| IBIS file was generated by Viper version: 2022.12.28
[IBIS Ver]   5.0
[Comment Char]   |_char
[File Name]   imxrt700_fowlp324_v1_2.ibs
[File Rev]   1.2
[Date]   Sat Oct 12 16:55:00 2024
[Source]   NXP Viper 2022.12.28
[Notes]
[Disclaimer] IMPORTANT NOTICE
  This information is provided on an AS IS basis and without warranty.
  IN NO EVENT SHALL NXP BE LIABLE FOR INCIDENTAL OR CONSEQUENTIAL
  DAMAGES ARISING FROM USE OF THIS INFORMATION. THIS DISCLAIMER OF
  WARRANTY EXTENDS TO THE USER OF THE INFORMATION, AND TO THEIR CUSTOMERS
  OR USERS OF PRODUCTS  AND IS IN LIEU OF ALL WARRANTIES WHETHER EXPRESS,
  IMPLIED, OR STATUTORY, INCLUDING IMPLIED WARRANTIES OF MERCHANTABILITY
  OR FITNESS FOR PARTICULAR PURPOSE.
  NXP does not represent or warrant that the information furnished
  hereunder is free of infringement of any third party patents,
  copyrights, trade secrets, or other intellectual property rights.
  NXP does not represent or warrant that the information is free of
  defect, or that it meets any particular standard, requirements or need
  of the user of the infomation or their customers.
  NXP reserves the right to change the information in this file
  without notice.
   http://www.nxp.com
[Copyright]   (C) Copyright NXP 2004 - 2024, All Rights Reserved.
|   RT700_324FOWLP_7p3x7p3
[Component]   RT700_324FOWLP_7p3x7p3
[Manufacturer]   NXP
[Package]
| variable   typ   min   max
R_pkg   0.26268   0.033092   0.85076
L_pkg   6.116e-10   1.144e-10   1.896e-09
C_pkg   3.384e-13   6.932e-14   8.387e-13
[Pin] signal_name   model_name   R_pin   L_pin   C_pin
A1   VSS   GND   NA   NA   NA
A2   MIPI_DSI_D1P   mipi   0.25124   1.051e-09 2.160e-13
A3   VSS   GND   NA   NA   NA
A4   MIPI_DSI_D0P   mipi   0.1054   3.119e-10 5.033e-13
A5   VSS   GND   NA   NA   NA
A6   PIO7_9   sd_mmc   0.12364   5.229e-10 1.490e-13
A7   VDDIO_0_4   POWER   NA   NA   NA
A8   VDD2_4   POWER   NA   NA   NA
A9   VDDIO_4   POWER   NA   NA   NA
A10   PIO4_5   sd_mmc   0.21739   8.630e-10 2.078e-13
A11   VSS   GND   NA   NA   NA
A12   VDDIO_4   POWER   NA   NA   NA
A13   VDD1V8   POWER   NA   NA   NA
A14   XTALINSYS   POWER   0.088384  3.992e-10 1.483e-13
A15   VCC18A   POWER   NA   NA   NA
A16   EUSB_DP   NC   0.28532   1.133e-09 1.995e-13
A17   EUSB_DM   NC   0.31827   1.299e-09 2.597e-13
A18   VSS   GND   NA   NA   NA
B1   MIPI_DSI_D1N   mipi   0.24947   1.078e-09 1.747e-13
B2   MIPI_DSI_CLKP   mipi   0.25909   9.091e-10 4.576e-13
B3   MIPI_DSI_CLKN   mipi   0.19446   7.269e-10 4.146e-13
B4   MIPI_DSI_D0N   mipi   0.068162  2.568e-10 2.976e-13
B5   VSS   GND   NA   NA   NA
B6   PIO7_0   sd_mmc   0.048221  3.150e-10 3.099e-13
B7   PIO7_6   sd_mmc   0.066435  1.963e-10 6.932e-14
B8   PIO7_7   sd_mmc   0.062862  3.240e-10 3.793e-13
B9   VDDIO_4   POWER   NA   NA   NA
B10   PIO4_10   sd_mmc   0.071774  2.949e-10 1.133e-13
B11   PIO4_11   sd_mmc   0.068127  3.496e-10 9.386e-14
B12   PIO4_8   sd_mmc   0.05942   3.399e-10 3.223e-13
B13   VDD1V8   POWER   NA   NA   NA
B14   XTALOUTSYS   POWER   0.040514  2.664e-10 2.477e-13
B15   VSS_EUSB   GND   NA   NA   NA
B16   VDD1V2_EUSB   POWER   NA   NA   NA
B17   VSS   GND   NA   NA   NA
B18   USB0_DP   NC   0.18414   6.632e-10 5.281e-13
C1   VDD2_3   POWER   NA   NA   NA
C2   VDD1V8_MIPI   POWER   NA   NA   NA
C3   PIO3_3   sd_mmc   0.20286   5.276e-10 2.379e-13
C4   VDD1V1_MIPI_CAP   POWER   NA   NA   NA
C5   PIO7_11   sd_mmc   0.063089  1.621e-10 3.202e-13
C6   PIO7_8   sd_mmc   0.13739   5.973e-10 3.845e-13
C7   PIO7_1   sd_mmc   0.11529   2.509e-10 1.486e-13
C8   PIO4_6   sd_mmc   0.30677   8.240e-10 4.205e-13
C9   PIO4_4   sd_mmc   0.27533   1.197e-09 5.637e-13
C10   PIO4_3   sd_mmc   0.19226   5.849e-10 3.079e-13
C11   PIO4_2   sd_mmc   0.14036   4.449e-10 2.674e-13
C12   PIO4_9   sd_mmc   0.070802  1.966e-10 1.609e-13
C13   PIO4_7   sd_mmc   0.20436   4.723e-10 3.672e-13
C14   VSSA_1   GND   NA   NA   NA
C15   PIO6_5   sd_mmc   0.11029   2.617e-10 1.678e-13
C16   USB0_VBUS_DETECT   POWER   0.043588  1.679e-10 1.579e-13
C17   VDDN_1   POWER   NA   NA   NA
C18   USB0_DM   NC   0.17462   7.141e-10 4.933e-13
D1   VDDIO_0_3   POWER   NA   NA   NA
D2   PIO3_2   sd_mmc   0.070338  2.788e-10 1.288e-13
D3   PIO2_15   gpiohv   0.20123   4.572e-10 2.051e-13
D4   PIO2_14   gpiohv   0.2838   6.011e-10 2.756e-13
D5   VSS   GND   NA   NA   NA
D6   PIO7_5   sd_mmc   0.13193   2.956e-10 1.907e-13
D7   VSS   GND   NA   NA   NA
D8   PIO4_0   sd_mmc   0.27396   9.004e-10 6.439e-13
D9   PIO4_1   sd_mmc   0.41757   9.862e-10 5.986e-13
D10   PIO4_20   sd_mmc   0.12261   3.165e-10 2.431e-13
D11   VSS   GND   NA   NA   NA
D12   PIO4_19   sd_mmc   0.31578   7.894e-10 4.764e-13
D13   VDDN_1   POWER   NA   NA   NA
D14   PIO6_4   sd_mmc   0.26259   5.271e-10 2.441e-13
D15   PIO6_7   sd_mmc   0.16583   3.647e-10 1.852e-13
D16   PIO6_0   sd_mmc   0.087097  2.313e-10 1.616e-13
D17   PIO6_1   sd_mmc   0.050073  3.030e-10 3.056e-13
D18   VDD3V3_USB   POWER   NA   NA   NA
E1   PIO3_0   sd_mmc   0.095738  4.384e-10 4.933e-13
E2   PIO3_1   sd_mmc   0.073279  1.998e-10 1.005e-13
E3   PIO2_12   gpiohv   0.18394   3.615e-10 3.051e-13
E4   PIO2_13   gpiohv   0.20149   3.491e-10 1.983e-13
E5   PIO7_10   sd_mmc   0.24125   5.709e-10 2.958e-13
E6   PIO7_4   sd_mmc   0.23404   4.870e-10 2.526e-13
E7   VSS   GND   NA   NA   NA
E8   PIO4_13   sd_mmc   0.389   9.169e-10 5.968e-13
E9   PIO4_18   sd_mmc   0.22306   4.870e-10 2.558e-13
E10   PIO4_15   sd_mmc   0.25504   5.203e-10 2.480e-13
E11   VSS   GND   NA   NA   NA
E12   PIO4_14   sd_mmc   0.33868   6.675e-10 4.529e-13
E13   PIO6_6   sd_mmc   0.31661   6.490e-10 4.919e-13
E14   PIO6_10   sd_mmc   0.2699   5.498e-10 2.719e-13
E15   VSS   GND   NA   NA   NA
E16   PIO5_6   sd_mmc   0.087982  1.970e-10 1.469e-13
E17   VDDIO_6   POWER   NA   NA   NA
E18   VDDIO_6   POWER   NA   NA   NA
F1   VDDIO_2   POWER   NA   NA   NA
F2   VDDIO_2   POWER   NA   NA   NA
F3   PIO2_11   gpiohv   0.10106   2.203e-10 1.988e-13
F4   VSS   GND   NA   NA   NA
F5   PIO2_10   gpiohv   0.27823   4.591e-10 4.477e-13
F6   PIO7_3   sd_mmc   0.33143   6.230e-10 3.363e-13
F7   PIO7_2   sd_mmc   0.32068   5.492e-10 3.128e-13
F8   PIO7_12   sd_mmc   0.33209   5.719e-10 4.215e-13
F9   PIO3_11   sd_mmc   0.70515   1.273e-09 5.479e-13
F10   PIO4_16   sd_mmc   0.3   6.269e-10 2.664e-13
F11   PIO4_12   sd_mmc   0.39643   7.821e-10 5.231e-13
F12   PIO4_17   sd_mmc   0.60927   1.113e-09 6.686e-13
F13   PIO6_3   sd_mmc   0.40489   8.103e-10 5.400e-13
F14   PIO6_11   sd_mmc   0.33137   7.151e-10 4.077e-13
F15   PIO6_9   sd_mmc   0.27209   6.555e-10 3.937e-13
F16   PIO5_4   sd_mmc   0.12263   2.688e-10 1.769e-13
F17   PIO5_10   sd_mmc   0.05928   3.299e-10 1.327e-13
F18   PIO5_3   sd_mmc   0.081794  4.401e-10 3.141e-13
G1   PIO2_3   gpiohv   0.10446   4.811e-10 1.576e-13
G2   PIO2_1   gpiohv   0.073468  3.339e-10 3.655e-13
G3   PIO2_4   gpiohv   0.041948  1.249e-10 1.778e-13
G4   PIO2_8   gpiohv   0.18251   2.949e-10 3.065e-13
G5   PIO2_9   gpiohv   0.27427   4.632e-10 3.930e-13
G6   PIO2_7   gpiohv   0.30133   5.353e-10 3.504e-13
G7   PIO3_8   sd_mmc   0.47105   9.259e-10 5.946e-13
G8   PIO3_9   sd_mmc   0.68953   1.205e-09 6.385e-13
G9   PIO3_10   sd_mmc   0.73021   1.279e-09 5.982e-13
G10   PIO6_12   sd_mmc   0.65976   1.205e-09 5.367e-13
G11   PIO6_2   sd_mmc   0.53692   1.044e-09 5.441e-13
G12   PIO7_24   sd_mmc   0.83454   1.421e-09 6.509e-13
G13   PIO6_8   sd_mmc   0.50655   1.022e-09 5.701e-13
G14   VSS   GND   NA   NA   NA
G15   VSS   GND   NA   NA   NA
G16   PIO5_5   sd_mmc   0.15144   4.193e-10 1.904e-13
G17   PIO5_11   sd_mmc   0.061307  2.373e-10 1.100e-13
G18   VSS   GND   NA   NA   NA
H1   VSS   GND   NA   NA   NA
H2   PIO2_0   gpiohv   0.078944  2.644e-10 8.475e-14
H3   PIO2_2   gpiohv   0.097119  2.358e-10 1.325e-13
H4   VSS   GND   NA   NA   NA
H5   VSS   GND   NA   NA   NA
H6   PIO2_6   gpiohv   0.33279   5.774e-10 4.006e-13
H7   PIO3_7   sd_mmc   0.62885   1.108e-09 7.148e-13
H8   VSS   GND   NA   NA   NA
H9   VSS   GND   NA   NA   NA
H10   VSS   GND   NA   NA   NA
H11   VSS   GND   NA   NA   NA
H12   PIO7_25   sd_mmc   0.71492   1.257e-09 5.744e-13
H13   PIO5_0   sd_mmc   0.25927   5.518e-10 3.250e-13
H14   PIO5_18   sd_mmc   0.26524   5.279e-10 2.383e-13
H15   PIO5_13   sd_mmc   0.18785   3.864e-10 2.251e-13
H16   PIO5_8   sd_mmc   0.20506   6.027e-10 2.558e-13
H17   PIO5_1   sd_mmc   0.48674   1.878e-09 4.866e-13
H18   PIO5_2   sd_mmc   0.29709   1.079e-09 2.137e-13
J1   PIO0_0   sd_mmc   0.13849   4.013e-10 4.956e-13
J2   PIO0_1   sd_mmc   0.090132  2.895e-10 1.213e-13
J3   PIO0_2   sd_mmc   0.10694   2.177e-10 1.417e-13
J4   PIO0_3   sd_mmc   0.21035   3.934e-10 2.174e-13
J5   PIO0_6   sd_mmc   0.2925   5.111e-10 2.939e-13
J6   PIO2_5   gpiohv   0.40854   6.791e-10 4.359e-13
J7   PIO3_6   sd_mmc   0.6273   1.093e-09 7.327e-13
J8   VSS   GND   NA   NA   NA
J9   VSS   GND   NA   NA   NA
J10   VSS   GND   NA   NA   NA
J11   VSS   GND   NA   NA   NA
J12   PIO8_26   gpio   0.75268   1.293e-09 6.117e-13
J13   PIO8_25   gpio   0.85076   1.583e-09 8.387e-13
J14   PIO5_15   sd_mmc   0.32094   7.312e-10 4.968e-13
J15   PIO5_16   sd_mmc   0.16604   4.852e-10 3.898e-13
J16   PIO5_9   sd_mmc   0.43442   1.046e-09 4.435e-13
J17   VDDIO_5   POWER   NA   NA   NA
J18   VDDIO_5   POWER   NA   NA   NA
K1   VDD2_2   POWER   NA   NA   NA
K2   VDD2_2   POWER   NA   NA   NA
K3   PIO0_5   sd_mmc   0.13395   3.094e-10 1.725e-13
K4   PIO0_4   sd_mmc   0.18653   3.791e-10 2.301e-13
K5   PIO0_7   sd_mmc   0.26742   5.072e-10 2.779e-13
K6   PIO3_4   sd_mmc   0.68031   1.153e-09 7.735e-13
K7   PIO3_5   sd_mmc   0.74255   1.238e-09 8.110e-13
K8   VSS   GND   NA   NA   NA
K9   VSS   GND   NA   NA   NA
K10   VSS   GND   NA   NA   NA
K11   VSS   GND   NA   NA   NA
K12   PIO8_27   gpio   0.65334   1.167e-09 5.593e-13
K13   PIO5_17   sd_mmc   0.3988   8.762e-10 4.868e-13
K14   PIO5_20   sd_mmc   0.35477   7.846e-10 4.492e-13
K15   PIO5_12   sd_mmc   0.23943   7.581e-10 3.363e-13
K16   PIO5_7   sd_mmc   0.35528   1.896e-09 4.801e-13
K17   PIO7_22   sd_mmc   0.059205  3.037e-10 3.223e-13
K18   PIO7_21   sd_mmc   0.088293  4.583e-10 3.666e-13
L1   PIO0_14   sd_mmc   0.11544   4.719e-10 1.283e-13
L2   PIO0_15   sd_mmc   0.066923  2.679e-10 1.285e-13
L3   PIO0_13   sd_mmc   0.094025  2.185e-10 1.477e-13
L4   PIO0_11   sd_mmc   0.16333   3.153e-10 2.063e-13
L5   PIO0_12   sd_mmc   0.26198   4.735e-10 3.649e-13
L6   PIO0_10   sd_mmc   0.34512   6.036e-10 4.896e-13
L7   PIO0_9   sd_mmc   0.41862   7.057e-10 5.931e-13
L8   VSS   GND   NA   NA   NA
L9   VSS   GND   NA   NA   NA
L10   VSS   GND   NA   NA   NA
L11   VSS   GND   NA   NA   NA
L12   PIO8_28   gpio   0.6211   1.126e-09 5.261e-13
L13   PIO5_19   sd_mmc   0.51582   1.825e-09 5.851e-13
L14   VSS   GND   NA   NA   NA
L15   VSS   GND   NA   NA   NA
L16   PIO7_18   sd_mmc   0.12585   2.973e-10 2.004e-13
L17   PIO7_17   sd_mmc   0.090307  5.404e-10 2.800e-13
L18   VDD2_0   POWER   NA   NA   NA
M1   VDDIO_0_2   POWER   NA   NA   NA
M2   PIO0_21   sd_mmc   0.064707  2.950e-10 3.688e-13
M3   PIO0_22   sd_mmc   0.099218  2.143e-10 9.874e-14
M4   VSS   GND   NA   NA   NA
M5   VSS   GND   NA   NA   NA
M6   PIO0_16   sd_mmc   0.34114   5.716e-10 4.635e-13
M7   PIO0_18   sd_mmc   0.51145   8.514e-10 4.167e-13
M8   PIO0_19   sd_mmc   0.53104   8.685e-10 5.914e-13
M9   PIO0_20   sd_mmc   0.65857   1.065e-09 7.339e-13
M10   PIO10_16   gpio   0.74355   1.222e-09 7.746e-13
M11   PIO10_15   gpio   0.70048   1.171e-09 6.645e-13
M12   PIO10_14   gpio   0.55175   1.004e-09 4.267e-13
M13   PIO5_14   sd_mmc   0.79821   1.373e-09 6.326e-13
M14   PIO7_15   sd_mmc   0.36129   7.960e-10 3.382e-13
M15   PIO7_16   sd_mmc   0.32048   8.596e-10 3.203e-13
M16   PIO8_7   gpio   0.11214   2.506e-10 1.514e-13
M17   PIO7_19   sd_mmc   0.12933   8.259e-10 2.940e-13
M18   PIO7_20   sd_mmc   0.14795   6.174e-10 1.476e-13
N1   PIO1_8   sd_mmc   0.19503   4.539e-10 2.024e-13
N2   PIO1_6   sd_mmc   0.16869   3.842e-10 5.100e-13
N3   PIO1_7   sd_mmc   0.223   5.144e-10 2.946e-13
N4   PIO0_31   sd_mmc   0.2088   3.681e-10 3.451e-13
N5   PIO1_0   sd_mmc   0.24232   4.470e-10 3.909e-13
N6   PIO0_17   sd_mmc   0.42268   7.407e-10 5.357e-13
N7   PMIC_MODE0   reset   0.71141   1.146e-09 5.418e-13
N8   PMIC_IRQN   gpio   0.61893   1.045e-09 4.873e-13
N9   PIO8_22   gpio   0.42049   7.439e-10 4.711e-13
N10   PIO10_17   gpio   0.72932   1.225e-09 7.125e-13
N11   PIO8_11   gpio   0.37601   6.916e-10 3.223e-13
N12   PIO8_10   gpio   0.38915   8.111e-10 3.420e-13
N13   PIO8_9   gpio   0.32668   6.628e-10 3.350e-13
N14   PIO7_23   sd_mmc   0.39583   9.471e-10 5.739e-13
N15   VSS   GND   NA   NA   NA
N16   PIO8_23   gpio   0.081719  4.063e-10 3.349e-13
N17   VDDIO_0_0   POWER   NA   NA   NA
N18   VDDIO_0_0   POWER   NA   NA   NA
P1   VSS   GND   NA   NA   NA
P2   VSS   GND   NA   NA   NA
P3   PIO1_14   sd_mmc   0.23155   4.677e-10 2.125e-13
P4   VSS   GND   NA   NA   NA
P5   PIO1_16   sd_mmc   0.22183   4.261e-10 2.054e-13
P6   PIO1_3   sd_mmc   0.28608   5.238e-10 3.286e-13
P7   PIO1_19   sd_mmc   0.41468   7.481e-10 3.525e-13
P8   VSS   GND   NA   NA   NA
P9   PIO8_19   gpio   0.32192   6.199e-10 3.699e-13
P10   PIO8_18   gpio   0.28934   5.565e-10 2.656e-13
P11   PIO8_12   gpio   0.33499   6.014e-10 4.740e-13
P12   VSS   GND   NA   NA   NA
P13   PIO8_30   gpio   0.32292   6.969e-10 3.223e-13
P14   PIO7_14   sd_mmc   0.35818   9.088e-10 3.617e-13
P15   PIO7_13   sd_mmc   0.28238   8.133e-10 3.868e-13
P16   PIO8_24   gpio   0.13641   3.373e-10 2.519e-13
P17   PIO10_3   gpio   0.10987   3.324e-10 3.455e-13
P18   PIO10_2   gpio   0.10227   5.228e-10 3.512e-13
R1   PIO1_12   sd_mmc   0.13573   5.705e-10 1.736e-13
R2   PIO1_11   sd_mmc   0.12126   5.284e-10 1.544e-13
R3   PIO1_13   sd_mmc   0.099978  2.118e-10 1.234e-13
R4   PIO1_17   sd_mmc   0.16732   3.573e-10 1.848e-13
R5   PIO1_18   sd_mmc   0.24552   4.548e-10 2.470e-13
R6   VSS   GND   NA   NA   NA
R7   PMIC_MODE1   reset   0.5507   8.938e-10 4.397e-13
R8   VSS   GND   NA   NA   NA
R9   PIO8_21   gpio   0.26922   5.156e-10 2.796e-13
R10   PIO8_14   gpio   0.26762   5.082e-10 2.516e-13
R11   PIO8_13   gpio   0.25   4.644e-10 2.232e-13
R12   VSS   GND   NA   NA   NA
R13   PIO8_31   gpio   0.33217   7.658e-10 3.659e-13
R14   VSS   GND   NA   NA   NA
R15   PIO10_4   gpio   0.12844   2.670e-10 2.052e-13
R16   PIO10_5   gpio   0.14117   3.322e-10 1.931e-13
R17   PIO10_0   gpio   0.085361  2.202e-10 3.274e-13
R18   VSS   GND   NA   NA   NA
T1   VDDIO_0_2   POWER   NA   NA   NA
T2   PIO1_10   sd_mmc   0.056962  2.821e-10 8.327e-14
T3   PIO1_5   sd_mmc   0.10396   2.135e-10 2.479e-13
T4   PIO1_4   sd_mmc   0.19114   3.228e-10 2.658e-13
T5   PIO1_9   sd_mmc   0.25441   4.057e-10 2.632e-13
T6   PIO1_15   sd_mmc   0.41215   7.309e-10 3.938e-13
T7   PIO1_2   sd_mmc   0.51869   9.147e-10 3.976e-13
T8   PIO8_20   gpio   0.28851   5.926e-10 3.523e-13
T9   PIO8_16   gpio   0.17418   3.140e-10 3.282e-13
T10   PIO8_15   gpio   0.096143  2.258e-10 2.472e-13
T11   PIO8_8   gpio   0.15183   3.244e-10 2.030e-13
T12   PIO8_1   gpio   0.15057   3.139e-10 1.938e-13
T13   PIO8_6   gpio   0.033092  1.144e-10 1.391e-13
T14   PIO10_6   gpio   0.11141   2.330e-10 1.541e-13
T15   PIO10_7   gpio   0.11856   2.511e-10 1.740e-13
T16   VREF_LDO   POWER   NA   NA   NA
T17   PIO10_1   gpio   0.089893  2.334e-10 4.163e-13
T18   PIO10_9   gpio   0.1209   3.477e-10 1.835e-13
U1   VDDIO_AO   POWER   NA   NA   NA
U2   VSS   GND   NA   NA   NA
U3   RESETN   reset   0.11889   2.360e-10 1.685e-13
U4   VDD1V8_AO   POWER   NA   NA   NA
U5   VDDN_0   POWER   NA   NA   NA
U6   VDD2_1   POWER   NA   NA   NA
U7   PMIC_I2C_SDA   gpio   0.1036   6.928e-10 4.221e-13
U8   PMIC_I2C_SCL   gpio   0.16925   9.938e-10 1.593e-13
U9   PIO8_17   gpio   0.22635   8.227e-10 5.004e-13
U10   VDD1   POWER   NA   NA   NA
U11   PIO8_2   gpio   0.10607   5.637e-10 4.373e-13
U12   PIO8_0   gpio   0.067902  2.438e-10 7.663e-14
U13   PIO8_5   gpio   0.067019  2.004e-10 3.449e-13
U14   VDDIO_0_1   POWER   NA   NA   NA
U15   PIO10_12   gpio   0.072742  3.968e-10 1.426e-13
U16   VREFH_ANA18   POWER   NA   NA   NA
U17   VREFL_ANA   POWER   NA   NA   NA
U18   PIO10_8   gpio   0.12168   3.775e-10 1.372e-13
V1   VSS   GND   NA   NA   NA
V2   XTALIN32KHZ   POWER   0.20791   1.009e-09 2.303e-13
V3   XTALOUT32KHZ   POWER   0.20324   6.472e-10 2.165e-13
V4   VDD1V8_AO   POWER   NA   NA   NA
V5   VSS   GND   NA   NA   NA
V6   VDD2_1   POWER   NA   NA   NA
V7   VDD1V8_DCDC   POWER   NA   NA   NA
V8   LX_DCDC   NC   0.034441  3.259e-10 3.584e-13
V9   VSS_DCDC   GND   NA   NA   NA
V10   VDD1   POWER   NA   NA   NA
V11   PIO8_3   gpio   0.11538   5.836e-10 1.100e-13
V12   VSS   GND   NA   NA   NA
V13   PIO8_4   gpio   0.11654   4.759e-10 2.414e-13
V14   VDDIO_0_1   POWER   NA   NA   NA
V15   PIO10_13   gpio   0.10932   5.018e-10 1.214e-13
V16   VDDA_1V8   POWER   NA   NA   NA
V17   VSSA_0   GND   NA   NA   NA
V18   VSSA_0   GND   NA   NA   NA
[Pin Mapping]   pulldown_ref   pullup_ref
A1   VSS   NC
A2   VSS   VDD1V8_MIPI
A3   VSS   NC
A4   VSS   VDD1V8_MIPI
A5   VSS   NC
A6   VSS   NC
A7   NC   VDDIO_0_4
A8   NC   VDD2_4
A9   NC   VDDIO_4
A10   VSS   VDDIO_4
A11   VSS   NC
A12   NC   VDDIO_4
A13   NC   VDD1V8
A14   NC   VDD1V8
A15   NC   VCC18A
A16   NC   NC
A17   NC   NC
A18   VSS   NC
B1   VSS   VDD1V8_MIPI
B2   VSS   VDD1V8_MIPI
B3   VSS   VDD1V8_MIPI
B4   VSS   VDD1V8_MIPI
B5   VSS   NC
B6   VSS   NC
B7   VSS   NC
B8   VSS   NC
B9   NC   VDDIO_4
B10   VSS   VDDIO_4
B11   VSS   VDDIO_4
B12   VSS   VDDIO_4
B13   NC   VDD1V8
B14   NC   VDD1V8
B15   VSS   NC
B16   NC   VDD1V2_EUSB
B17   VSS   NC
B18   NC   NC
C1   NC   VDD2_3
C2   NC   VDD1V8_MIPI
C3   VSS   NC
C4   NC   VDD1V1_MIPI_CAP
C5   VSS   NC
C6   VSS   NC
C7   VSS   NC
C8   VSS   VDDIO_4
C9   VSS   VDDIO_4
C10   VSS   VDDIO_4
C11   VSS   VDDIO_4
C12   VSS   VDDIO_4
C13   VSS   VDDIO_4
C14   VSSA_1   NC
C15   VSS   VDDIO_6
C16   NC   VDD3V3_USB
C17   NC   VDDN_1
C18   NC   NC
D1   NC   VDDIO_0_3
D2   VSS   NC
D3   VSS   VDDIO_2
D4   VSS   VDDIO_2
D5   VSS   NC
D6   VSS   NC
D7   VSS   NC
D8   VSS   VDDIO_4
D9   VSS   VDDIO_4
D10   VSS   VDDIO_4
D11   VSS   NC
D12   VSS   VDDIO_4
D13   NC   VDDN_1
D14   VSS   VDDIO_6
D15   VSS   VDDIO_6
D16   VSS   VDDIO_6
D17   VSS   VDDIO_6
D18   NC   VDD3V3_USB
E1   VSS   NC
E2   VSS   NC
E3   VSS   VDDIO_2
E4   VSS   VDDIO_2
E5   VSS   NC
E6   VSS   NC
E7   VSS   NC
E8   VSS   VDDIO_4
E9   VSS   VDDIO_4
E10   VSS   VDDIO_4
E11   VSS   NC
E12   VSS   VDDIO_4
E13   VSS   VDDIO_6
E14   VSS   VDDIO_6
E15   VSS   NC
E16   VSS   VDDIO_5
E17   NC   VDDIO_6
E18   NC   VDDIO_6
F1   NC   VDDIO_2
F2   NC   VDDIO_2
F3   VSS   VDDIO_2
F4   VSS   NC
F5   VSS   VDDIO_2
F6   VSS   NC
F7   VSS   NC
F8   VSS   NC
F9   VSS   NC
F10   VSS   VDDIO_4
F11   VSS   VDDIO_4
F12   VSS   VDDIO_4
F13   VSS   VDDIO_6
F14   VSS   VDDIO_6
F15   VSS   VDDIO_6
F16   VSS   VDDIO_5
F17   VSS   VDDIO_5
F18   VSS   VDDIO_5
G1   VSS   VDDIO_2
G2   VSS   VDDIO_2
G3   VSS   VDDIO_2
G4   VSS   VDDIO_2
G5   VSS   VDDIO_2
G6   VSS   VDDIO_2
G7   VSS   NC
G8   VSS   NC
G9   VSS   NC
G10   VSS   VDDIO_6
G11   VSS   VDDIO_6
G12   VSS   NC
G13   VSS   VDDIO_6
G14   VSS   NC
G15   VSS   NC
G16   VSS   VDDIO_5
G17   VSS   VDDIO_5
G18   VSS   NC
H1   VSS   NC
H2   VSS   VDDIO_2
H3   VSS   VDDIO_2
H4   VSS   NC
H5   VSS   NC
H6   VSS   VDDIO_2
H7   VSS   NC
H8   VSS   NC
H9   VSS   NC
H10   VSS   NC
H11   VSS   NC
H12   VSS   NC
H13   VSS   VDDIO_5
H14   VSS   VDDIO_5
H15   VSS   VDDIO_5
H16   VSS   VDDIO_5
H17   VSS   VDDIO_5
H18   VSS   VDDIO_5
J1   VSS   NC
J2   VSS   NC
J3   VSS   NC
J4   VSS   NC
J5   VSS   NC
J6   VSS   VDDIO_2
J7   VSS   NC
J8   VSS   NC
J9   VSS   NC
J10   VSS   NC
J11   VSS   NC
J12   VSS   NC
J13   VSS   NC
J14   VSS   VDDIO_5
J15   VSS   VDDIO_5
J16   VSS   VDDIO_5
J17   NC   VDDIO_5
J18   NC   VDDIO_5
K1   NC   VDD2_2
K2   NC   VDD2_2
K3   VSS   NC
K4   VSS   NC
K5   VSS   NC
K6   VSS   NC
K7   VSS   NC
K8   VSS   NC
K9   VSS   NC
K10   VSS   NC
K11   VSS   NC
K12   VSS   NC
K13   VSS   VDDIO_5
K14   VSS   VDDIO_5
K15   VSS   VDDIO_5
K16   VSS   VDDIO_5
K17   VSS   NC
K18   VSS   NC
L1   VSS   NC
L2   VSS   NC
L3   VSS   NC
L4   VSS   NC
L5   VSS   NC
L6   VSS   NC
L7   VSS   NC
L8   VSS   NC
L9   VSS   NC
L10   VSS   NC
L11   VSS   NC
L12   VSS   NC
L13   VSS   VDDIO_5
L14   VSS   NC
L15   VSS   NC
L16   VSS   NC
L17   VSS   NC
L18   NC   VDD2_0
M1   NC   VDDIO_0_2
M2   VSS   NC
M3   VSS   NC
M4   VSS   NC
M5   VSS   NC
M6   VSS   NC
M7   VSS   NC
M8   VSS   NC
M9   VSS   NC
M10   VSS   NC
M11   VSS   NC
M12   VSS   NC
M13   VSS   VDDIO_5
M14   VSS   NC
M15   VSS   NC
M16   VSS   NC
M17   VSS   NC
M18   VSS   NC
N1   VSS   NC
N2   VSS   NC
N3   VSS   NC
N4   VSS   NC
N5   VSS   NC
N6   VSS   NC
N7   VSS   VDDIO_AO
N8   VSS   VDDIO_AO
N9   VSS   NC
N10   VSS   NC
N11   VSS   NC
N12   VSS   NC
N13   VSS   NC
N14   VSS   NC
N15   VSS   NC
N16   VSS   NC
N17   NC   VDDIO_0_0
N18   NC   VDDIO_0_0
P1   VSS   NC
P2   VSS   NC
P3   VSS   NC
P4   VSS   NC
P5   VSS   NC
P6   VSS   NC
P7   VSS   NC
P8   VSS   NC
P9   VSS   NC
P10   VSS   NC
P11   VSS   NC
P12   VSS   NC
P13   VSS   NC
P14   VSS   NC
P15   VSS   NC
P16   VSS   NC
P17   VSS   NC
P18   VSS   NC
R1   VSS   NC
R2   VSS   NC
R3   VSS   NC
R4   VSS   NC
R5   VSS   NC
R6   VSS   NC
R7   VSS   VDDIO_AO
R8   VSS   NC
R9   VSS   NC
R10   VSS   NC
R11   VSS   NC
R12   VSS   NC
R13   VSS   NC
R14   VSS   NC
R15   VSS   NC
R16   VSS   NC
R17   VSS   NC
R18   VSS   NC
T1   NC   VDDIO_0_2
T2   VSS   NC
T3   VSS   NC
T4   VSS   NC
T5   VSS   NC
T6   VSS   NC
T7   VSS   NC
T8   VSS   NC
T9   VSS   NC
T10   VSS   NC
T11   VSS   NC
T12   VSS   NC
T13   VSS   NC
T14   VSS   NC
T15   VSS   NC
T16   NC   VDDA_1V8
T17   VSS   NC
T18   VSS   NC
U1   NC   VDDIO_AO
U2   VSS   NC
U3   VSS   VDDIO_AO
U4   NC   VDD1V8_AO
U5   NC   VDDN_0
U6   NC   VDD2_1
U7   VSS   NC
U8   VSS   NC
U9   VSS   NC
U10   NC   VDD1
U11   VSS   NC
U12   VSS   NC
U13   VSS   NC
U14   NC   VDDIO_0_1
U15   VSS   NC
U16   NC   VDDA_1V8
U17   NC   VDDA_1V8
U18   VSS   NC
V1   VSS   NC
V2   NC   VDDIO_AO
V3   NC   VDDIO_AO
V4   NC   VDD1V8_AO
V5   VSS   NC
V6   NC   VDD2_1
V7   NC   VDD1V8_DCDC
V8   NC   NC
V9   VSS_DCDC   NC
V10   NC   VDD1
V11   VSS   NC
V12   VSS   NC
V13   VSS   NC
V14   NC   VDDIO_0_1
V15   VSS   NC
V16   NC   VDDA_1V8
V17   VSSA_0   NC
V18   VSSA_0   NC
[Diff Pin]  inv_pin  vdiff  tdelay_typ tdelay_min tdelay_max
A2   B1   NA   NA   NA   NA
A4   B4   NA   NA   NA   NA
B2   B3   NA   NA   NA   NA
|*   Model Selector   *
[Model Selector] gpio
io_crdrobe1dse0sre0   Derated range in cont mode, 5mA drive strength, without slew rate
io_crdrobe1dse0sre1   Derated range in cont mode, 5mA drive strength, with slew rate
io_crdrobe1dse1sre0   Derated range in cont mode, 10mA drive strength, without slew rate
io_crdrobe1dse1sre1   Derated range in cont mode, 10mA drive strength, with slew rate
io_crdr2obe1dse0sre0   Derated2 range in cont mode, 5mA drive strength, without slew rate
io_crdr2obe1dse0sre1   Derated2 range in cont mode, 5mA drive strength, with slew rate
io_crdr2obe1dse1sre0   Derated2 range in cont mode, 10mA drive strength, without slew rate
io_crdr2obe1dse1sre1   Derated2 range in cont mode, 10mA drive strength, with slew rate
io_lrobe1dse0sre0   low range mode, 5mA drive strength, without slew rate
io_lrobe1dse0sre1   low range mode, 5mA drive strength, with slew rate
io_lrobe1dse1sre0   low range mode, 10mA drive strength, without slew rate
io_lrobe1dse1sre1   low range mode, 10mA drive strength, with slew rate
[Model Selector] gpiohv
io_crnrobe1dse0sre0   Normal range in cont mode, 5mA drive strength, without slew rate
io_crnrobe1dse0sre1   Normal range in cont mode, 5mA drive strength, with slew rate
io_crnrobe1dse1sre0   Normal range in cont mode, 10mA drive strength, without slew rate
io_crnrobe1dse1sre1   Normal range in cont mode, 10mA drive strength, with slew rate
io_crdrobe1dse0sre0   Derated range in cont mode, 5mA drive strength, without slew rate
io_crdrobe1dse0sre1   Derated range in cont mode, 5mA drive strength, with slew rate
io_crdrobe1dse1sre0   Derated range in cont mode, 10mA drive strength, without slew rate
io_crdrobe1dse1sre1   Derated range in cont mode, 10mA drive strength, with slew rate
io_crdr2obe1dse0sre0   Derated2 range in cont mode, 5mA drive strength, without slew rate
io_crdr2obe1dse0sre1   Derated2 range in cont mode, 5mA drive strength, with slew rate
io_crdr2obe1dse1sre0   Derated2 range in cont mode, 10mA drive strength, without slew rate
io_crdr2obe1dse1sre1   Derated2 range in cont mode, 10mA drive strength, with slew rate
io_hrobe1dse0sre0   high range mode, 5mA drive strength, without slew rate
io_hrobe1dse0sre1   high range mode, 5mA drive strength, with slew rate
io_hrobe1dse1sre0   high range mode, 10mA drive strength, without slew rate
io_hrobe1dse1sre1   high range mode, 10mA drive strength, with slew rate
io_lrobe1dse0sre0   low range mode, 5mA drive strength, without slew rate
io_lrobe1dse0sre1   low range mode, 5mA drive strength, with slew rate
io_lrobe1dse1sre0   low range mode, 10mA drive strength, without slew rate
io_lrobe1dse1sre1   low range mode, 10mA drive strength, with slew rate
io_crnrobe1dse0sre0_5pct   Narrow range in cont mode, 5mA drive strength, without slew rate
io_crnrobe1dse0sre1_5pct   Narrow range in cont mode, 5mA drive strength, with slew rate
io_crnrobe1dse1sre0_5pct   Narrow range in cont mode, 10mA drive strength, without slew rate
io_crnrobe1dse1sre1_5pct   Narrow range in cont mode, 10mA drive strength, with slew rate
io_hrobe1dse0sre0_5pct   Narrow range in high range mode, 5mA drive strength, without slew rate
io_hrobe1dse0sre1_5pct   Narrow range in high range mode, 5mA drive strength, with slew rate
io_hrobe1dse1sre0_5pct   Narrow range in high range mode, 10mA drive strength, without slew rate
io_hrobe1dse1sre1_5pct   Narrow range in high range mode, 10mA drive strength, with slew rate
[Model Selector] mipi
MIPI_HS   MIPI DSI High Speed Mode
MIPI_LP   MIPI DSI Low Power Mode
[Model Selector] reset
io_rst_crdrobe1dse0sre0   Derated voltage range in cont mode, 5mA current drive strength, without slew rate
io_rst_crdrobe1dse0sre1   Derated voltage range in cont mode, 5mA current drive strength, with slew rate
io_rst_crdrobe1dse1sre0   Derated voltage range in cont mode, 10mA current drive strength, without slew rate
io_rst_crdrobe1dse1sre1   Derated voltage range in cont mode, 10mA current drive strength, with slew rate
io_rst_crdr2obe1dse0sre0   Derated2 voltage range in cont mode, 5mA current drive strength, without slew rate
io_rst_crdr2obe1dse0sre1   Derated2 voltage range in cont mode, 5mA current drive strength, with slew rate
io_rst_crdr2obe1dse1sre0   Derated2 voltage range in cont mode, 10mA current drive strength, without slew rate
io_rst_crdr2obe1dse1sre1   Derated2 voltage range in cont mode, 10mA current drive strength, with slew rate
io_rst_lrobe1dse0sre0   low range mode, 5mA current drive strength, without slew rate
io_rst_lrobe1dse0sre1   low range mode, 5mA current drive strength, with slew rate
io_rst_lrobe1dse1sre0   low range mode, 10mA current drive strength, without slew rate
io_rst_lrobe1dse1sre1   low range mode, 10mA current drive strength, with slew rate
[Model Selector] sd_mmc
io_nvldro0drz0   Normal voltage level DRIVE1=0 DRIVE0=0 1.8v voltage domain function mode with 100ohm transmitter drive
io_nvldro0drz1   Normal voltage level DRIVE1=0 DRIVE0=1 1.8v voltage domain function mode with 66ohm transmitter drive
io_nvldro1drz0   Normal voltage level DRIVE1=1 DRIVE0=0 1.8v voltage domain function mode with 50ohm transmitter drive
io_nvldro1drz1   Normal voltage level DRIVE1=1 DRIVE0=1 1.8v voltage domain function mode with 33ohm transmitter drive
io_lvldro0drz0   low voltage level DRIVE1=0 DRIVE0=0 1.2v voltage domain function mode with 100ohm transmitter drive
io_lvldro0drz1   low voltage level DRIVE1=0 DRIVE0=1 1.2v voltage domain function mode with 66ohm transmitter drive
io_lvldro1drz0   low voltage level DRIVE1=1 DRIVE0=0 1.2v voltage domain function mode with 50ohm transmitter drive
io_lvldro1drz1   low voltage level DRIVE1=1 DRIVE0=1 1.2v voltage domain function mode with 33ohm transmitter drive
| End [Component] RT700_324FOWLP_7p3x7p3
| Models and submodels in the file (50): MIPI_HS (Output), MIPI_LP (I/O), io_crdr2obe1dse0sre0 (I/O), io_crdr2obe1dse0sre1 (I/O), io_crdr2obe1dse1sre0 (I/O), io_crdr2obe1dse1sre1 (I/O), io_crdrobe1dse0sre0 (I/O), io_crdrobe1dse0sre1 (I/O), io_crdrobe1dse1sre0 (I/O), io_crdrobe1dse1sre1 (I/O), io_crnrobe1dse0sre0 (I/O), io_crnrobe1dse0sre0_5pct (I/O), io_crnrobe1dse0sre1 (I/O), io_crnrobe1dse0sre1_5pct (I/O), io_crnrobe1dse1sre0 (I/O), io_crnrobe1dse1sre0_5pct (I/O), io_crnrobe1dse1sre1 (I/O), io_crnrobe1dse1sre1_5pct (I/O), io_hrobe1dse0sre0 (I/O), io_hrobe1dse0sre0_5pct (I/O), io_hrobe1dse0sre1 (I/O), io_hrobe1dse0sre1_5pct (I/O), io_hrobe1dse1sre0 (I/O), io_hrobe1dse1sre0_5pct (I/O), io_hrobe1dse1sre1 (I/O), io_hrobe1dse1sre1_5pct (I/O), io_lrobe1dse0sre0 (I/O), io_lrobe1dse0sre1 (I/O), io_lrobe1dse1sre0 (I/O), io_lrobe1dse1sre1 (I/O), io_lvldro0drz0 (I/O), io_lvldro0drz1 (I/O), io_lvldro1drz0 (I/O), io_lvldro1drz1 (I/O), io_nvldro0drz0 (I/O), io_nvldro0drz1 (I/O), io_nvldro1drz0 (I/O), io_nvldro1drz1 (I/O), io_rst_crdr2obe1dse0sre0 (I/O), io_rst_crdr2obe1dse0sre1 (I/O), io_rst_crdr2obe1dse1sre0 (I/O), io_rst_crdr2obe1dse1sre1 (I/O), io_rst_crdrobe1dse0sre0 (I/O), io_rst_crdrobe1dse0sre1 (I/O), io_rst_crdrobe1dse1sre0 (I/O), io_rst_crdrobe1dse1sre1 (I/O), io_rst_lrobe1dse0sre0 (I/O), io_rst_lrobe1dse0sre1 (I/O), io_rst_lrobe1dse1sre0 (I/O), io_rst_lrobe1dse1sre1 (I/O)
